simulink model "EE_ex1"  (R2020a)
settings: Solver=VariableStepAuto  StartTime=0.0  StopTime=50  RelTol=1e-3

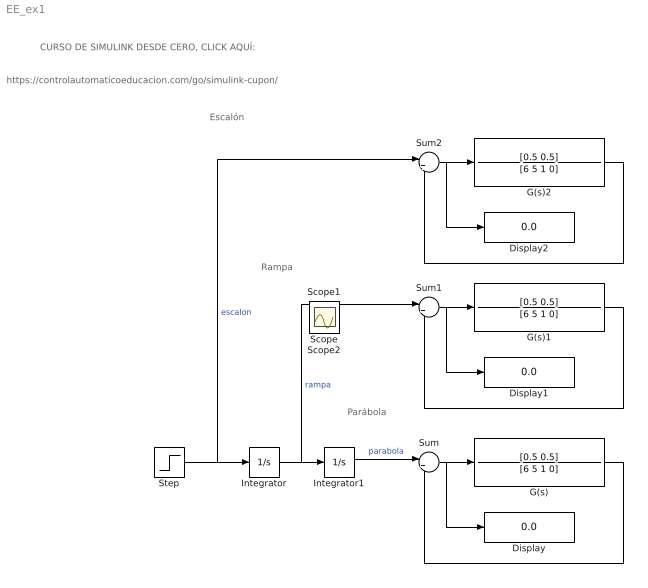
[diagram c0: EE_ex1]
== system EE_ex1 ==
  note: https://controlautomaticoeducacion.com/go/simulink-cupon/
  note: Escalón
  note: Rampa
  note: Parábola
  note: CURSO DE SIMULINK DESDE CERO, CLICK AQUÍ:
  Display : Display
  Display1 : Display
  Display2 : Display
  G(s) : TransferFcn  Numerator=[0.5 0.5]  Denominator=[6 5 1 0]
  G(s)1 : TransferFcn  Numerator=[0.5 0.5]  Denominator=[6 5 1 0]
  G(s)2 : TransferFcn  Numerator=[0.5 0.5]  Denominator=[6 5 1 0]
  Integrator : Integrator
  Integrator1 : Integrator
  Step : Step  Time=0  After=3  SampleTime=0
  Sum : Sum  Inputs=|+-
  Sum1 : Sum  Inputs=|+-
  Sum2 : Sum  Inputs=|+-
  Scope : Scope
  Scope1 : Scope
  Scope2 : Scope
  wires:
  Sum/1 -> Display/1, G(s)/1
  Integrator/1 -> Sum1/1, Integrator1/1  "rampa"
  Step/1 -> Sum2/1, Integrator/1  "escalon"
  Integrator1/1 -> Sum/1  "parabola"
  G(s)/1 -> Sum/2
  G(s)1/1 -> Sum1/2
  Sum1/1 -> G(s)1/1, Display1/1
  Sum2/1 -> Display2/1, G(s)2/1
  G(s)2/1 -> Sum2/2
